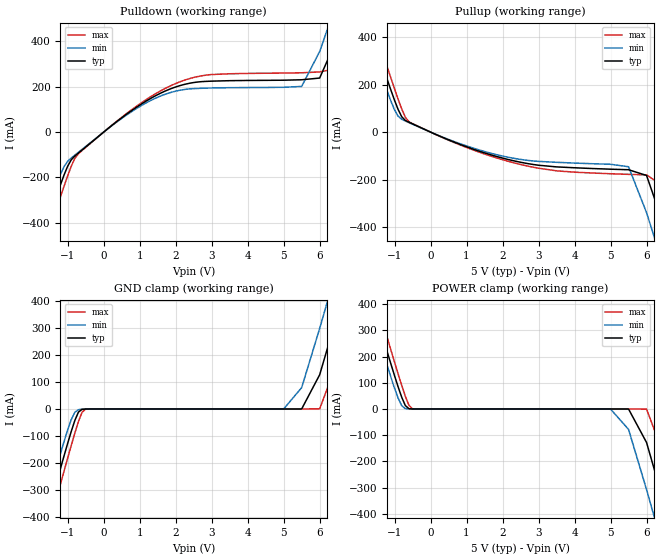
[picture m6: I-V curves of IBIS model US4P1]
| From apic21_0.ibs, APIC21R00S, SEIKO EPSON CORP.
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[Model]   US4P1
Model_type   I/O
Polarity   Non-Inverting
Vinh=2.0V
Vinl=0.8V
|   typ   min   max
C_comp   0   NA   NA
|   typ   min   max
[Voltage range]   5.0   4.5   5.5
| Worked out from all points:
|   slope of the pulldown table from 0 to 0.75 V, typ, clamps not added: 8.17 ohm
|   slope of the pullup table from 0 to 0.75 V, typ, clamps not added: 15.7 ohm
|   GND clamp passes 1 mA (typ) near -0.57 V on its own axis
|   POWER clamp passes 1 mA (typ) near -0.60 V on its own axis
[Pulldown]
|   Voltage   I(typ)   I(min)   I(max)
-10V      -4.642A    -4.562A    -4.722A
-1.9V     -566.9mA   -507mA     -628.2mA
-1.6V     -420.5mA   -363.5mA   -479.7mA
-1.1V     -189mA     -152.1mA   -238.3mA
-700mV    -92.09mA   -89mA      -95.27mA
1.7V      180.1mA    166mA      191.6mA
2.9V      223.7mA    193.9mA    252mA
5.5V      230.5mA    201.2mA    261.2mA
6V        238.1mA    355mA      265.1mA
6.5V      417.6mA    582.1mA    280.6mA
7V        648.7mA    815.9mA    482.3mA
10V       2.086A     2.248A     1.923A
[Pullup]
|   Voltage   I(typ)   I(min)   I(max)
-10V      4.425A     4.351A     4.501A
-1.9V     543.7mA    486.7mA    601.8mA
-1.6V     403.5mA    348.5mA    460mA
-1V       134.3mA    94.05mA    182.5mA
-700mV    49.18mA    46.55mA    62.69mA
-500mV    34.58mA    33.18mA    35.77mA
2.5V      -127.1mA   -115.2mA   -136.4mA
5.5V      -158.7mA   -146.1mA   -178.2mA
6V        -182.8mA   -339.7mA   -180.3mA
6.5V      -401.8mA   -579.5mA   -231.7mA
7V        -645.5mA   -825.1mA   -465.2mA
10V       -2.147A    -2.323A    -1.97A
[GND_clamp]
|   Voltage   I(typ)   I(min)   I(max)
-10V      -4.641A    -4.561A    -4.722A
-1.7V     -464.4mA   -404.1mA   -526mA
-1.5V     -366.4mA   -307.5mA   -426.8mA
-1.4V     -317.7mA   -259.7mA   -377.4mA
-900mV    -83.36mA   -39.48mA   -135.4mA
-500mV    -283.5uA   -329.1uA   -653.3uA
5V        319.4pA    38.04uA    -10uA
5.5V      47.76uA    79.28mA    300.3pA
6V        127.1mA    299.3mA    664.9uA
6.5V      354.7mA    531.1mA    178.7mA
7V        589.3mA    766.1mA    411.3mA
10V       2.021A     2.194A     1.847A
[POWER_clamp]
|   Voltage   I(typ)   I(min)   I(max)
-10V      4.425A     4.35A      4.5A
-1.8V     495mA      437.8mA    553.3mA
-1.6V     401.3mA    345.2mA    458.5mA
-1.5V     354.7mA    299.3mA    411.4mA
-900mV    84.31mA    41.36mA    133.6mA
-500mV    47.76uA    38.04uA    664.9uA
5V        -100uA     -329.1uA   -100uA
5.5V      -283.5uA   -77.93mA   -110uA
6V        -127.9mA   -307.3mA   -653.1uA
6.5V      -366.3mA   -550.6mA   -182.6mA
7V        -612.6mA   -797.4mA   -426.8mA
10V       -2.117A    -2.297A    -1.935A
[Ramp]
|   V_typ   V_min   V_max
dV/dt_r   3.00/2.993e-10   2.70/3.124e-10   3.30/2.897e-10
dV/dt_f   3.00/2.758e-10   2.70/2.860e-10   3.30/2.723e-10
R_load = 5000ohm
